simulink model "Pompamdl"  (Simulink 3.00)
settings: Solver=ode45  StartTime=0.0  StopTime=10.0  RelTol=1e-6  AbsTol=1e-6
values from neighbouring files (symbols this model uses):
  bm = Ic0*KI/Wmax    [Pompa.m]
  Ia0 = 0    [Pompa.m]
  Jm = 9.2775e-006    (= 9.2775e-06)    [Pompa.m]
  Km = 10    [Esempio.m]    (also in Pompa.m = 0.00651965811966)
  La = 60*10^-6    (= 6e-05)    [Pompa.m]
  Ra = Vn/Imax    (= 0.128205128205)    [Pompa.m]
  Tcsim = 1*msec    (= 0.001)    [Pompa.m]
  Wme0 = 0    [Pompa.m]
undefined symbols (not defined in the file or in its folder): al_0, K0, Kp
libraries: simulink3 x2

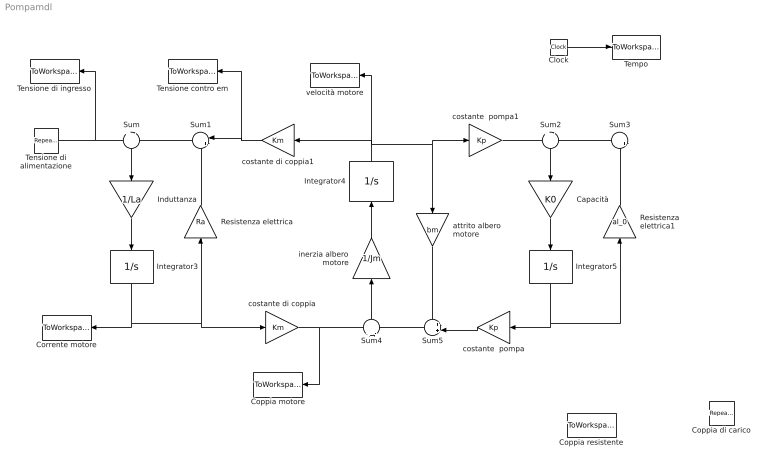
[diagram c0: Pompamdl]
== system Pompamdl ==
  Capacità : Gain  Orientation=down  Gain=K0  SaturateOnIntegerOverflow=on
  Clock : Clock
  Coppia motore : ToWorkspace  VariableName=Cm  SampleTime=Tcsim  SaveFormat=Matrix
  Coppia resistente : ToWorkspace  VariableName=Cr  SampleTime=Tcsim  SaveFormat=Matrix
  Coppia di carico : simulink3/Sources/Repeating Sequence  Orientation=left  rep_seq_t=TABTEMPI  rep_seq_y=TABCR
  Corrente motore : ToWorkspace  VariableName=Ia  SampleTime=Tcsim  SaveFormat=Matrix
  Induttanza : Gain  Orientation=down  Gain=1/La  SaturateOnIntegerOverflow=on
  Integrator3 : Integrator  Orientation=down  ExternalReset=none  InitialConditionSource=internal  InitialCondition=Ia0  LimitOutput=off  UpperSaturationLimit=inf  LowerSaturationLimit=-inf  ShowSaturationPort=off  ShowStatePort=off  AbsoluteTolerance=auto
  Integrator4 : Integrator  Orientation=up  ExternalReset=none  InitialConditionSource=internal  InitialCondition=Wme0  LimitOutput=off  UpperSaturationLimit=inf  LowerSaturationLimit=-inf  ShowSaturationPort=off  ShowStatePort=off  AbsoluteTolerance=auto
  Integrator5 : Integrator  Orientation=down  ExternalReset=none  InitialConditionSource=internal  InitialCondition=Ia0  LimitOutput=off  UpperSaturationLimit=inf  LowerSaturationLimit=-inf  ShowSaturationPort=off  ShowStatePort=off  AbsoluteTolerance=auto
  Resistenza elettrica : Gain  Orientation=up  Gain=Ra  SaturateOnIntegerOverflow=on
  Resistenza elettrica1 : Gain  Orientation=up  Gain=al_0  SaturateOnIntegerOverflow=on
  Sum : Sum  Orientation=down  Inputs=+|-  SaturateOnIntegerOverflow=on
  Sum1 : Sum  Orientation=left  Inputs=|++  SaturateOnIntegerOverflow=on
  Sum2 : Sum  Orientation=down  Inputs=+|-  SaturateOnIntegerOverflow=on
  Sum3 : Sum  Orientation=left  Inputs=|++  SaturateOnIntegerOverflow=on
  Sum4 : Sum  Orientation=up  Inputs=+|-  SaturateOnIntegerOverflow=on
  Sum5 : Sum  Orientation=left  Inputs=++|  SaturateOnIntegerOverflow=on
  Tempo : ToWorkspace  VariableName=t  SampleTime=Tcsim  SaveFormat=Matrix
  Tensione contro em : ToWorkspace  VariableName=Vcem  SampleTime=Tcsim  SaveFormat=Matrix
  Tensione di ingresso : ToWorkspace  VariableName=Vi  SampleTime=Tcsim  SaveFormat=Matrix
  Tensione di alimentazione : simulink3/Sources/Repeating Sequence  rep_seq_t=TABTEMPI  rep_seq_y=TABVIN
  attrito albero motore : Gain  Orientation=down  Gain=bm  SaturateOnIntegerOverflow=on
  costante  pompa1 : Gain  Gain=Kp  SaturateOnIntegerOverflow=on
  costante di coppia : Gain  Gain=Km  SaturateOnIntegerOverflow=on
  costante di coppia1 : Gain  Orientation=left  Gain=Km  SaturateOnIntegerOverflow=on
  costante  pompa : Gain  Orientation=left  Gain=Kp  SaturateOnIntegerOverflow=on
  inerzia albero motore : Gain  Orientation=up  Gain=1/Jm  SaturateOnIntegerOverflow=on
  velocità motore : ToWorkspace  VariableName=Wm  SampleTime=Tcsim  SaveFormat=Matrix
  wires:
  Tensione di alimentazione/1 -> Sum/1, Tensione di ingresso/1
  Sum/1 -> Induttanza/1
  Induttanza/1 -> Integrator3/1
  Clock/1 -> Tempo/1
  Integrator3/1 -> Corrente motore/1, costante di coppia/1, Resistenza elettrica/1
  Sum1/1 -> Sum/2
  Resistenza elettrica/1 -> Sum1/2
  costante di coppia1/1 -> Sum1/1, Tensione contro em/1
  costante di coppia/1 -> Sum4/1, Coppia motore/1
  inerzia albero motore/1 -> Integrator4/1
  Integrator4/1 -> velocità motore/1, attrito albero motore/1, costante  pompa1/1, costante di coppia1/1
  Sum4/1 -> inerzia albero motore/1
  Sum5/1 -> Sum4/2
  attrito albero motore/1 -> Sum5/1
  costante  pompa/1 -> Sum5/2
  costante  pompa1/1 -> Sum2/1
  Sum2/1 -> Capacità/1
  Capacità/1 -> Integrator5/1
  Integrator5/1 -> Resistenza elettrica1/1, costante  pompa/1
  Sum3/1 -> Sum2/2
  Resistenza elettrica1/1 -> Sum3/2
  ? -> Sum3/1
